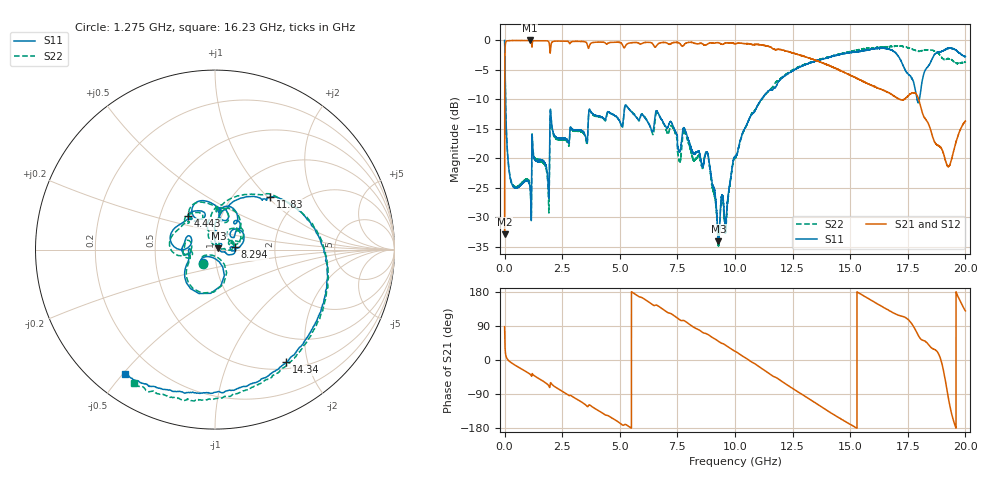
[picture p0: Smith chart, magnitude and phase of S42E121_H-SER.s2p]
!{S42E121}
!Johanson Technology Inc.
!www.johansontechnology.com
!Test Board Conditions:
!Substrate Type  RO4350B
!Substrate Thickness  50 mil
!Substrate Dk  3.66
!TL Type: GCPW
!TL Trace Width  60 mil
!TL Gap  10 mil
!Electrode orientation  Horizontal
!DUT TOPOLOGY	SERIES
!Mounting Pad LxW  14x55 mil
! Created Wed Nov 25 21:57:37 2020
# khz S ma R 50
! 2 Port Network Data from SP1.SP block
! freq  magS11  angS11  magS21  angS21  magS12  angS12  magS22  angS22
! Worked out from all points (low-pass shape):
!   20001 points, 300 kHz to 20 GHz, reference 50 ohm
!   highest |S21| = -0.02 dB at 1.1 GHz (marker M1); lowest = -32.9 dB at 300 kHz (marker M2)
!   |S21| within 3 dB of the highest: 13.21 MHz to 13.23 GHz (13.22 GHz wide, 200 % of centre); 13.24326 GHz to 13.24331 GHz (58.66 kHz wide, 0.000443 % of centre)
!   lowest |S11| = -34.0 dB at 9.282 GHz (marker M3), VSWR 1.04, Z = 51.9 + j0.699 ohm
!   |S11| at or under -10 dB: 39.63 MHz to 11.14 GHz (11.1 GHz wide, 199 % of centre); 17.9 GHz to 18 GHz (96.97 MHz wide, 0.54 % of centre)
!   |S22| runs from -34.9 to 0.0 dB; largest |S21 - S12| = 0.012
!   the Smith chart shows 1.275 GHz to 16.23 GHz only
!   S11 on the Smith chart (normalised r, x): 1.275 GHz: 0.86, -0.13; 4.443 GHz: 0.69, +0.28; 8.294 GHz: 1.25, +0.03; 11.83 GHz: 1.45, +1.04; 14.34 GHz: 0.59, -1.66; 16.23 GHz: 0.10, -0.51
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300  0.9967 -1.4  0.02273 87.9  0.02276 88.6  0.9941 -1.4
113300  0.1216 -88.1  0.9904 2.8  0.991 2.8  0.1226 -87.9
350300  0.059 -101.7  0.9964 -9.6  0.9963 -9.6  0.05972 -101.0
1100300  0.05718 -128.5  0.9976 -37.3  0.9967 -37.3  0.05932 -125.6
1275300  0.1012 -133.2  0.9922 -41.1  0.9919 -41.1  0.1037 -128.5
1848300  0.07611 -145.9  0.9898 -63.3  0.99 -63.3  0.07118 -151.3
3334300  0.1725 155.2  0.9786 -110.7  0.9789 -110.7  0.1682 164.1
4443300  0.2411 128.7  0.9309 -145.9  0.9299 -145.9  0.235 136.1
6667300  0.2414 61.3  0.9351 142.5  0.9319 142.4  0.2375 59.8
8294300  0.1122 6.9  0.9382 83.5  0.9369 83.7  0.09858 23.3
8803300  0.1113 -7.8  0.9288 68.3  0.9291 68.2  0.1091 10.3
9282300  0.01988 19.8  0.9535 49.1  0.9557 49.0  0.01854 38.2
1.00003e7  0.1033 86.9  0.9363 22.9  0.937 23.0  0.1015 107.0
1.18293e7  0.4261 43.6  0.8374 -47.8  0.8365 -47.7  0.4522 40.4
1.33343e7  0.6516 -16.8  0.695 -107.2  0.6992 -107.2  0.6578 -17.0
1.43413e7  0.743 -57.7  0.5821 -146.2  0.5879 -146.2  0.749 -54.2
1.62263e7  0.8561 -126.0  0.3922 146.4  0.3904 146.9  0.8705 -121.4
1.66673e7  0.8405 -141.6  0.3615 131.5  0.3531 131.9  0.8877 -136.8
1.79513e7  0.2964 -164.6  0.3252 65.4  0.3259 66.4  0.8077 -174.9
1.85213e7  0.6729 -162.6  0.1667 32.3  0.1672 33.0  0.8265 167.8
1.92473e7  0.8531 155.3  0.0856 -95.3  0.08528 -95.8  0.7025 146.6
2e7  0.7292 124.8  0.2068 129.6  0.207 130.2  0.6525 123.5
